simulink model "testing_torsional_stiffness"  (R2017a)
settings: Solver=ode23t  StartTime=0.0  StopTime=10  MaxStep=0.02  RelTol=1e-3  AbsTol=1e-3  EnableMultiTasking=on
undefined symbols (not defined in the file): damping, radius_a, radius_b
libraries: fl_lib x10, nesl_utility x3

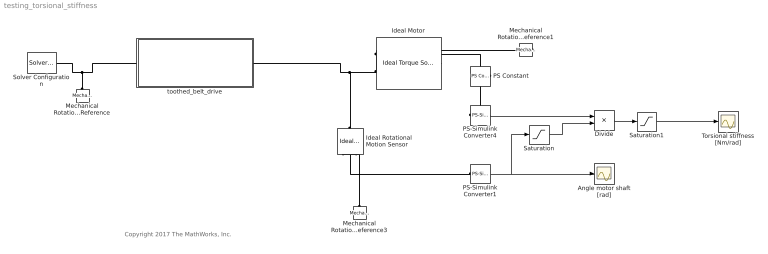
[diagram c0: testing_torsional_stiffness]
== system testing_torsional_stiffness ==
  note: Copyright 2017 The MathWorks, Inc.
  Angle motor shaft [rad] : Scope
  Divide : Product  Inputs=*/
  Ideal Motor : fl_lib/Mechanical/Mechanical Sources/Ideal Torque Source
  Ideal Rotational Motion Sensor : fl_lib/Mechanical/Mechanical Sensors/Ideal Rotational Motion Sensor  offset=0 rad
  Mechanical Rotational Reference : fl_lib/Mechanical/Rotational Elements/Mechanical Rotational Reference
  Mechanical Rotational Reference1 : fl_lib/Mechanical/Rotational Elements/Mechanical Rotational Reference
  Mechanical Rotational Reference3 : fl_lib/Mechanical/Rotational Elements/Mechanical Rotational Reference
  PS Constant : fl_lib/Physical Signals/Sources/PS Constant  constant=1
  PS-Simulink Converter1 : nesl_utility/PS-Simulink Converter  PhysicalDomain=network_engine_domain  SubClassName=ps_output  LeftPortType=input  RightPortType=output  PseudoPeriodic=off  Frequencies=[]  Unit=rad  AffineConversion=off
  PS-Simulink Converter4 : nesl_utility/PS-Simulink Converter  PhysicalDomain=network_engine_domain  SubClassName=ps_output  LeftPortType=input  RightPortType=output  PseudoPeriodic=off  Frequencies=[]  Unit=N*m  AffineConversion=off
  Saturation : Saturate  UpperLimit=inf  LowerLimit=1e-10
  Saturation1 : Saturate  UpperLimit=1e6  LowerLimit=0
  Solver Configuration : nesl_utility/Solver Configuration  PhysicalDomain=network_engine_domain  SubClassName=solver  LeftPortType=input  RightPortType=generic  Accelerate=off  Tones=[]  Harmonics=[]  SimulateNoise=off  Profile=off  UseLocalSampling=off  EnableSwitchedLinearOptims=on  FrequencyDomain=off  UseCCode=off  RelTol=0.001  AbsTol=1e-06  MinStep=1e-09  ToWorkspace=off  RevertToSquareIcSolve=off  NumHomotopyIterations=100  PhasorMode=off  PhasorModeNumHarmonics=1  OverrideAbsTol=off  DoDC=off  ResidualTolerance=1e-09  UseLocalSolver=off  LocalSolverChoice=NE_BACKWARD_EULER_ADVANCER  LocalSolverSampleTime=0.001  DoFixedCost=off  MaxNonlinIter=3  MaxModeIter=2  LinearAlgebra=Sparse  DelaysMemoryBudget=1024  AutomaticFiltering=on  FilteringTimeConstant=0.001
  Torsional stiffness [Nm/rad] : Scope
  toothed_belt_drive : Subsystem
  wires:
  PS-Simulink Converter1/1 -> Saturation/1, Angle motor shaft [rad]/1
  Divide/1 -> Saturation1/1
  PS-Simulink Converter4/1 -> Divide/1
  Saturation/1 -> Divide/2
  Saturation1/1 -> Torsional stiffness [Nm/rad]/1
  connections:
  Ideal Motor/RConn2 -- Mechanical Rotational Reference1/LConn1
  PS-Simulink Converter1/LConn1 -- Ideal Rotational Motion Sensor/RConn3
  Mechanical Rotational Reference3/LConn1 -- Ideal Rotational Motion Sensor/RConn1
  PS Constant/RConn1 -- PS-Simulink Converter4/LConn1 -- Ideal Motor/RConn1
  Mechanical Rotational Reference/LConn1 -- Solver Configuration/RConn1 -- toothed_belt_drive/LConn1
  Ideal Rotational Motion Sensor/LConn1 -- toothed_belt_drive/RConn1 -- Ideal Motor/LConn1

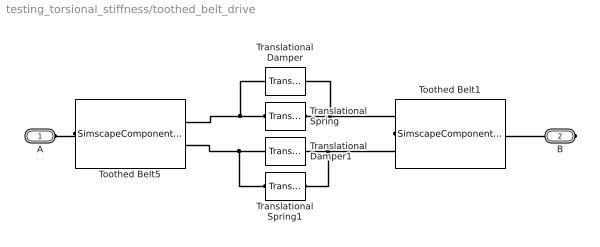
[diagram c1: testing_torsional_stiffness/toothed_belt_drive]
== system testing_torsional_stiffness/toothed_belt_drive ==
  Toothed Belt1 : SimscapeComponentBlock  SourceFile=toothed_pulley  ComponentPath=toothed_pulley  ComponentVariants=toothed_pulley  ComponentVariantNames=toothed_pulley  ClassName=toothed_pulley  SchemaVersion=1  R=radius_b mm  b_pulley=mu_visc_b N*m/(rad/s)  pulley_inertia=inertia_b kg*m^2  initial_velocity=0 rad/s  t_specify=off  t_priority=None  t=0 N*m  t_nominal_specify=off  t_nominal_unit=N*m  t_nominal_value=1  fA_specify=off  fA_priority=None  fA=0 N  fA_nominal_specify=off  fA_nominal_unit=N  fA_nominal_value=1  fB_specify=off  fB_priority=None  fB=0 N  fB_nominal_specify=off  fB_nominal_unit=N  fB_nominal_value=1
  Toothed Belt5 : SimscapeComponentBlock  SourceFile=toothed_pulley  ComponentPath=toothed_pulley  ComponentVariants=toothed_pulley  ComponentVariantNames=toothed_pulley  ClassName=toothed_pulley  SchemaVersion=1  R=radius_a mm  b_pulley=mu_visc_a N*m/(rad/s)  pulley_inertia=inertia_a kg*m^2  initial_velocity=0 rad/s  t_specify=off  t_priority=None  t=0 N*m  t_nominal_specify=off  t_nominal_unit=N*m  t_nominal_value=1  fA_specify=off  fA_priority=None  fA=0 N  fA_nominal_specify=off  fA_nominal_unit=N  fA_nominal_value=1  fB_specify=off  fB_priority=None  fB=0 N  fB_nominal_specify=off  fB_nominal_unit=N  fB_nominal_value=1
  Translational Damper : fl_lib/Mechanical/Translational Elements/Translational Damper  D=damping N/(m/s)  v_specify=off  v_priority=None  v=0 m/s  v_nominal_specify=off  v_nominal_unit=m/s  v_nominal_value=1  f_specify=off  f_priority=None  f=0 N  f_nominal_specify=off  f_nominal_unit=N  f_nominal_value=1
  Translational Damper1 : fl_lib/Mechanical/Translational Elements/Translational Damper  D=damping N/(m/s)  v_specify=off  v_priority=None  v=0 m/s  v_nominal_specify=off  v_nominal_unit=m/s  v_nominal_value=1  f_specify=off  f_priority=None  f=0 N  f_nominal_specify=off  f_nominal_unit=N  f_nominal_value=1
  Translational Spring : fl_lib/Mechanical/Translational Elements/Translational Spring  spr_rate=stiffness N/mm  v_specify=off  v_priority=None  v=0 m/s  v_nominal_specify=off  v_nominal_unit=m/s  v_nominal_value=1  f_specify=on  f_priority=High  f=tension N  f_nominal_specify=off  f_nominal_unit=N  f_nominal_value=1  x_specify=on  x_priority=None  x=0 m  x_nominal_specify=off  x_nominal_unit=m  x_nominal_value=1
  Translational Spring1 : fl_lib/Mechanical/Translational Elements/Translational Spring  spr_rate=stiffness N/mm  v_specify=off  v_priority=None  v=0 m/s  v_nominal_specify=off  v_nominal_unit=m/s  v_nominal_value=1  f_specify=on  f_priority=High  f=tension N  f_nominal_specify=off  f_nominal_unit=N  f_nominal_value=1  x_specify=on  x_priority=None  x=0 m  x_nominal_specify=off  x_nominal_unit=m  x_nominal_value=1
  A : PMIOPort  Port=1  Side=Left
  B : PMIOPort  Port=2  Side=Right
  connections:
  Translational Spring1/RConn1 -- Translational Damper1/RConn1 -- Toothed Belt1/RConn1
  Translational Spring1/LConn1 -- Translational Damper1/LConn1 -- Toothed Belt5/RConn2
  Translational Spring/RConn1 -- Translational Damper/RConn1 -- Toothed Belt1/RConn2
  Translational Spring/LConn1 -- Translational Damper/LConn1 -- Toothed Belt5/RConn1
  Toothed Belt5/LConn1 -- A/RConn1
  Toothed Belt1/LConn1 -- B/RConn1
